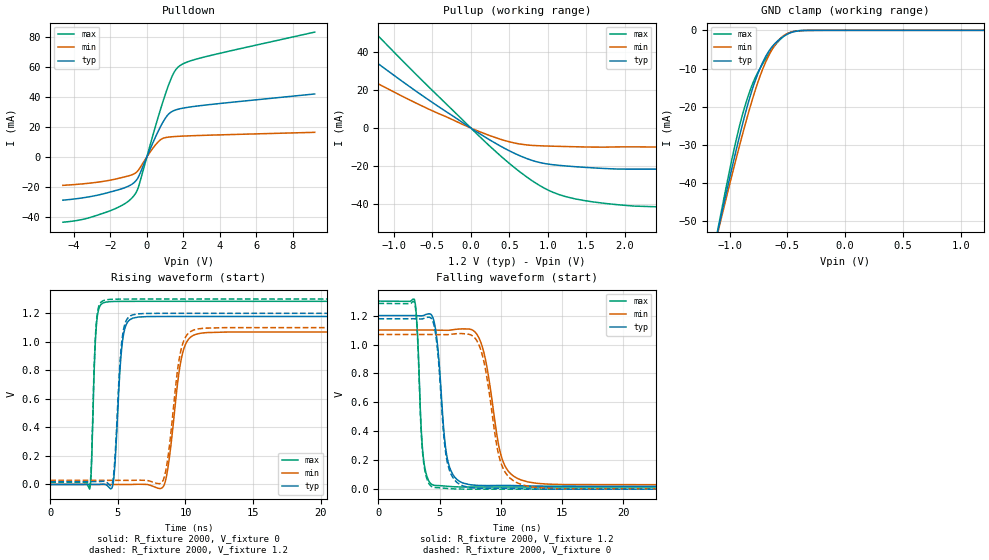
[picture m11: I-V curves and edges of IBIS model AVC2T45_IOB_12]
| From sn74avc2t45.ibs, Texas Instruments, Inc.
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[Model]   AVC2T45_IOB_12
Model_type  I/O
Vinl=0.42
Vinh=0.78
Enable   Active-High
Vref =   0
Rref =   2000
Cref =   15p
Vmeas =   0.6
| variable   typ   min   max
C_comp   5.29pF   4.69pF   5.84pF
| C_pullup   5.78pF   3.90pF   7.84pF
| C_pulldown   5.33pF   4.75pF   7.04pF
| C_tri-state   5.29pF   4.69pF   5.84pF
[Temperature Range]   40   100   -40
| Ambient temperature   25   85   -40
[Voltage range]   1.2   NA   NA
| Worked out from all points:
|   slope of the pulldown table from 0 to 0.18 V, typ, clamps not added: 34.6 ohm
|   slope of the pullup table from 0 to 0.18 V, typ, clamps not added: 38.6 ohm
|   GND clamp passes 1 mA (typ) near -0.50 V on its own axis
|   rising waveform, R_fixture 2000, V_fixture 0: 20-80 % time 428ps typ, 795ps min, 259ps max; typ from 0 V to 1.18 V
|   falling waveform, R_fixture 2000, V_fixture 1.2: 20-80 % time 671ps typ, 1.22ns min, 400ps max; typ from 1.2 V to 0.02 V
|   rising waveform, R_fixture 2000, V_fixture 1.2: 20-80 % time 422ps typ, 772ps min, 257ps max; typ from 0.02 V to 1.2 V
|   falling waveform, R_fixture 2000, V_fixture 0: 20-80 % time 670ps typ, 1.21ns min, 398ps max; typ from 1.18 V to 0 V
[GND Clamp]
| AVC2T45_IOB_12
|   Voltage   I(typ)   I(min)   I(max)
-4.6V     -597.8mA   -546.6mA   -662.5mA
-1.095V   -51.41mA   -51.9mA    -50.81mA
-1.07V    -47.97mA   -48.78mA   -46.93mA
-940mV    -30.76mA   -33.04mA   -28.1mA
-840mV    -18.99mA   -21.8mA    -17.13mA
-775mV    -12.84mA   -15.28mA   -12.1mA
-695mV    -7.204mA   -8.735mA   -7.744mA
-615mV    -3.665mA   -4.111mA   -4.191mA
-545mV    -1.809mA   -1.649mA   -1.862mA
-465mV    -549.4uA   -452.3uA   -430.6uA
-360mV    -50.53uA   -51.18uA   -21.62uA
1.2V      708.7pA    34.41nA    62.33pA
[Pulldown]
| AVC2T45_IOB_12
|   Voltage   I(typ)   I(min)   I(max)
-4.6V     -28.79mA   -18.92mA   -43.46mA
-3.415V   -27.06mA   -17.81mA   -41.32mA
-2.03V    -23.44mA   -15.52mA   -35.94mA
-1.165V   -20.28mA   -13.12mA   -30.82mA
-680mV    -16.87mA   -11.13mA   -25.38mA
-435mV    -12.68mA   -8.327mA   -19.06mA
440mV     12.38mA    7.543mA    19.04mA
955mV     24.67mA    12.69mA    39.57mA
1.42V     30.53mA    13.49mA    54.64mA
1.79V     32.04mA    13.78mA    60.61mA
3.17V     34.51mA    14.41mA    66.63mA
9.2V      41.96mA    16.4mA     83.17mA
[Pullup]
| AVC2T45_IOB_12
|   Voltage   I(typ)   I(min)   I(max)
-4.6V     40.24mA    7.956mA    186.3mA
-4.08V    45.4mA     8.808mA    167.8mA
-3.73V    53.62mA    9.647mA    154.2mA
-2.685V   79.31mA    16.98mA    111.4mA
-2.57V    75.87mA    21.96mA    106.5mA
-2.565V   75.72mA    49.42mA    106.3mA
-1.845V   53.66mA    37.03mA    75.82mA
-1.36V    38.76mA    26.71mA    55.3mA
575mV     -13.51mA   -7.977mA   -21.19mA
1.01V     -19.08mA   -9.527mA   -32.92mA
1.455V    -20.71mA   -9.971mA   -38.21mA
9.2V      -28.28mA   -12.48mA   -52.65mA
[Ramp]
| AVC2T45_IOB_12
| variable   typ   min   max
dV/dt_r   0.72/4.41E-10   0.66/8.17E-10   0.79/2.78E-10
dV/dt_f   0.72/6.81E-10   0.65/1.23E-09   0.78/4.08E-10
R_load = 2000
[Rising Waveform]
| AVC2T45_IOB_12
R_fixture =   2000
C_fixture =   0
L_fixture =   0
V_fixture =   0
V_fixture_min = 0
V_fixture_max = 0
|   Time   V(typ)   V(min)   V(max)
0s        18.11nV    102nV      416.8pV
2.91ns    9.581uV    1.031uV    -33.05mV
3.395ns   -92.06uV   -4.294uV   1.097V
3.97ns    2.12mV     6.869uV    1.275V
4.65ns    7.185mV    4.809uV    1.283V
5.32ns    987.8mV    -49.17uV   1.284V
6.115ns   1.167V     163.8uV    1.284V
8.43ns    1.178V     -1.782mV   1.284V
10.77ns   1.178V     1.053V     1.284V
40ns      1.178V     1.069V     1.284V
[Falling Waveform]
| AVC2T45_IOB_12
R_fixture =   2000
C_fixture =   0
L_fixture =   0
V_fixture =   1.2
V_fixture_min = 1.1
V_fixture_max = 1.3
|   Time   V(typ)   V(min)   V(max)
0s        1.2V       1.1V       1.3V
2.94ns    1.2V       1.1V       1.308V
3.64ns    1.2V       1.1V       237.4mV
4.445ns   1.185V     1.1V       29.3mV
5.59ns    225.3mV    1.098V     20.24mV
6.875ns   43.07mV    1.108V     15.07mV
8.33ns    25.65mV    1.02V      14.54mV
10.03ns   25.88mV    227.8mV    14.51mV
11.62ns   23.68mV    64.2mV     14.5mV
40ns      20.14mV    28.75mV    14.5mV
[Rising Waveform]
| AVC2T45_IOB_12
R_fixture =   2000
C_fixture =   0
L_fixture =   0
V_fixture =   1.2
V_fixture_min = 1.1
V_fixture_max = 1.3
|   Time   V(typ)   V(min)   V(max)
0s        20.14mV    28.74mV    14.5mV
2.91ns    20.14mV    28.74mV    -17.64mV
3.39ns    20.05mV    28.74mV    1.115V
3.98ns    22.08mV    28.75mV    1.291V
4.64ns    32.95mV    28.75mV    1.299V
5.305ns   1.016V     28.7mV     1.3V
6.09ns    1.189V     28.87mV    1.3V
8.36ns    1.2V       31.45mV    1.3V
10.64ns   1.2V       1.084V     1.3V
40ns      1.2V       1.1V       1.3V
[Falling Waveform]
| AVC2T45_IOB_12
R_fixture =   2000
C_fixture =   0
L_fixture =   0
V_fixture =   0
V_fixture_min = 0
V_fixture_max = 0
|   Time   V(typ)   V(min)   V(max)
0s        1.178V     1.069V     1.284V
2.94ns    1.178V     1.069V     1.291V
3.63ns    1.178V     1.069V     227mV
4.4ns     1.169V     1.069V     15.74mV
5.575ns   204.5mV    1.068V     5.195mV
6.875ns   23.06mV    1.075V     469.8uV
8.265ns   5.716mV    984.2mV    39.56uV
9.925ns   5.785mV    201.2mV    8.367uV
11.55ns   3.354mV    36.06mV    2.44uV
40ns      76.74nV    5.607uV    23.63nV
